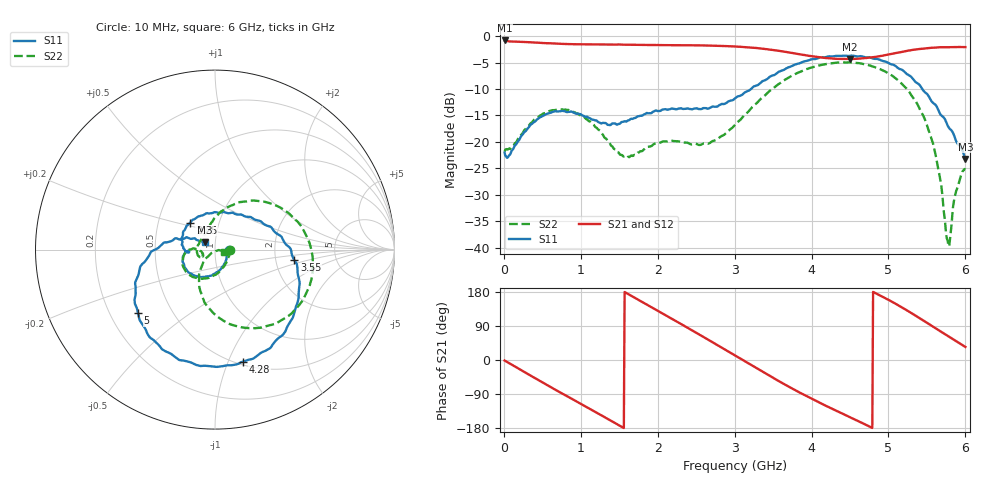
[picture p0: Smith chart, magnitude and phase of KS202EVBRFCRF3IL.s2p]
!Agilent Technologies,N5230A,MY45001650,A.07.50.48
!Agilent N5230A: A.07.50.48
!Date: Monday, June 12, 2017 12:52:11
!Correction: S11(Full 2 Port(1,2))
!S21(Full 2 Port(1,2))
!S12(Full 2 Port(1,2))
!S22(Full 2 Port(1,2))
!S2P File: Measurements: S11, S21, S12, S22:
# Hz S  dB  R 50
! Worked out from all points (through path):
!   600 points, 10 MHz to 6 GHz, reference 50 ohm
!   highest |S21| = -0.82 dB at 10 MHz (marker M1); lowest = -4.4 dB at 4.5 GHz (marker M2)
!   group delay of S21, straight-line fit = 314 ps
!   lowest |S11| = -23.2 dB at 6 GHz (marker M3), VSWR 1.15, Z = 44.6 + j3.59 ohm
!   |S11| at or under -10 dB: start of sweep to 3.213 GHz; 5.439 GHz to end of sweep
!   |S22| runs from -39.7 to -5.0 dB; largest |S21 - S12| = 0.0025
!   S11 on the Smith chart (normalised r, x): 10 MHz: 1.17, -0.00; 2.25 GHz: 0.73, +0.23; 3.55 GHz: 2.54, -0.37; 4.28 GHz: 0.53, -1.13; 5 GHz: 0.32, -0.33; 6 GHz: 0.89, +0.07
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1e7  -22.04 -1.4  -0.82 -1.4  -0.81 -1.4  -21.84 -0.5
2.6e8  -18.27 -80.2  -1.11 -30.9  -1.10 -30.9  -17.95 -79.3
5.4e8  -14.85 -125.5  -1.34 -63.6  -1.33 -63.6  -14.52 -122.9
1.01e9  -14.89 -168.7  -1.55 -116.8  -1.55 -116.7  -15.04 -168.9
1.51e9  -16.55 -175.5  -1.59 -173.8  -1.59 -173.7  -22.43 -171.5
2.01e9  -14.17 158.8  -1.69 128.9  -1.69 129.0  -20.26 -157.9
2.25e9  -13.82 132.6  -1.72 101.2  -1.72 101.3  -19.89 -177.8
2.6e9  -13.61 90.8  -1.77 60.2  -1.77 60.4  -20.30 139.8
3.01e9  -11.73 44.8  -1.97 11.4  -1.97 11.6  -16.70 99.3
3.26e9  -9.47 22.0  -2.22 -18.4  -2.22 -18.3  -13.02 78.2
3.55e9  -7.02 -7.5  -2.74 -52.8  -2.74 -52.7  -9.31 52.9
4.01e9  -4.36 -51.0  -3.81 -103.1  -3.80 -103.1  -5.90 11.5
4.28e9  -3.83 -75.9  -4.25 -130.0  -4.26 -130.0  -5.11 -11.7
4.5e9  -3.74 -95.5  -4.35 -151.0  -4.35 -151.1  -4.97 -30.0
5e9  -5.09 -140.4  -3.48 158.7  -3.48 158.7  -7.05 -74.0
5.01e9  -5.17 -141.5  -3.45 157.7  -3.45 157.6  -7.13 -75.0
5.25e9  -7.27 -165.6  -2.76 129.7  -2.76 129.6  -10.15 -99.3
5.5e9  -10.92 171.9  -2.28 98.3  -2.29 98.3  -16.85 -125.4
5.65e9  -14.05 163.4  -2.12 79.0  -2.12 78.9  -25.21 -134.9
5.77e9  -16.93 155.0  -2.10 63.7  -2.10 63.7  -38.75 -76.4
5.88e9  -19.88 151.0  -2.07 49.7  -2.07 49.7  -29.32 -8.7
6e9  -23.25 144.4  -2.08 34.4  -2.09 34.4  -25.26 -15.3
